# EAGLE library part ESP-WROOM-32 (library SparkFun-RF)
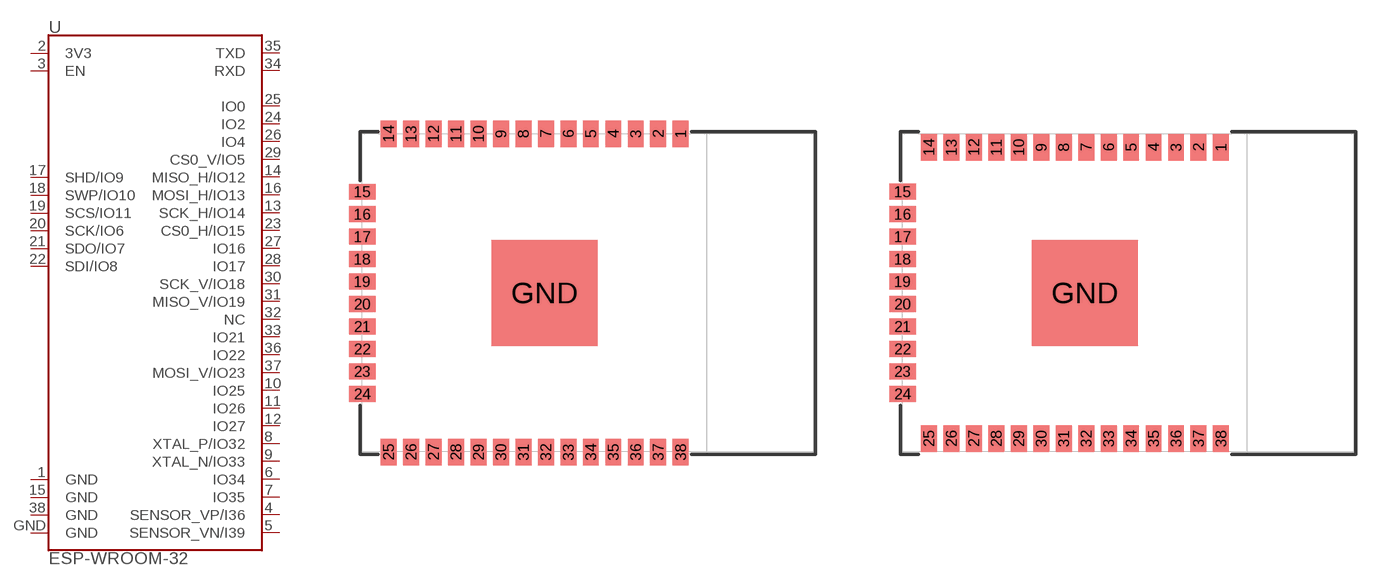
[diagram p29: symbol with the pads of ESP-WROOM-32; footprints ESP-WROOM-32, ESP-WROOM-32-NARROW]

Designator prefix U

## ESP-WROOM-32 (PROD_ID: IC-13849)  [ESP-WROOM-32]
1  GND
2  3V3
3  EN
4  SENSOR_VP/I36
5  SENSOR_VN/I39
6  IO34
7  IO35
8  XTAL_P/IO32
9  XTAL_N/IO33
10  IO25
11  IO26
12  IO27
13  SCK_H/IO14
14  MISO_H/IO12
15  GND
16  MOSI_H/IO13
17  SHD/IO9
18  SWP/IO10
19  SCS/IO11
20  SCK/IO6
21  SDO/IO7
22  SDI/IO8
23  CS0_H/IO15
24  IO2
25  IO0
26  IO4
27  IO16
28  IO17
29  CS0_V/IO5
30  SCK_V/IO18
31  MISO_V/IO19
32  NC
33  IO21
34  RXD
35  TXD
36  IO22
37  MOSI_V/IO23
38  GND
GND  GND

## ESP-WROOM-32NARROW (PROD_ID: IC-13849)  [ESP-WROOM-32-NARROW]
Pads as for ESP-WROOM-32

## Footprint ESP-WROOM-32 (pad centres in mm)
smd 0.9 x 1.5: 1 7.7,9; 2 6.43,9; 3 5.16,9; 4 3.89,9; 5 2.62,9; 6 1.35,9; 7 0.08,9; 8 -1.19,9; 9 -2.46,9; 10 -3.73,9; 11 -5,9; 12 -6.27,9; 13 -7.54,9; 14 -8.81,9; 25 -8.81,-9; 26 -7.54,-9; 27 -6.27,-9; 28 -5,-9; 29 -3.73,-9; 30 -2.46,-9; 31 -1.19,-9; 32 0.08,-9; 33 1.35,-9; 34 2.62,-9; 35 3.89,-9; 36 5.16,-9; 37 6.43,-9; 38 7.7,-9
smd 1.5 x 0.9: 15 -10.3,5.715; 16 -10.3,4.445; 17 -10.3,3.175; 18 -10.3,1.905; 19 -10.3,0.635; 20 -10.3,-0.635; 21 -10.3,-1.905; 22 -10.3,-3.175; 23 -10.3,-4.445; 24 -10.3,-5.715
smd 6 x 6: GND 0,0

## Footprint ESP-WROOM-32-NARROW (pad centres in mm)
smd 0.9 x 1.5: 1 6.43,8.238; 2 5.16,8.238; 3 3.89,8.238; 4 2.62,8.238; 5 1.35,8.238; 6 0.08,8.238; 7 -1.19,8.238; 8 -2.46,8.238; 9 -3.73,8.238; 10 -5,8.238; 11 -6.27,8.238; 12 -7.54,8.238; 13 -8.81,8.238; 14 -10.08,8.238; 25 -10.08,-8.238; 26 -8.81,-8.238; 27 -7.54,-8.238; 28 -6.27,-8.238; 29 -5,-8.238; 30 -3.73,-8.238; 31 -2.46,-8.238; 32 -1.19,-8.238; 33 0.08,-8.238; 34 1.35,-8.238; 35 2.62,-8.238; 36 3.89,-8.238; 37 5.16,-8.238; 38 6.43,-8.238
smd 1.5 x 0.9: 15 -11.57,5.715; 16 -11.57,4.445; 17 -11.57,3.175; 18 -11.57,1.905; 19 -11.57,0.635; 20 -11.57,-0.635; 21 -11.57,-1.905; 22 -11.57,-3.175; 23 -11.57,-4.445; 24 -11.57,-5.715
smd 6 x 6: GND -1.27,0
